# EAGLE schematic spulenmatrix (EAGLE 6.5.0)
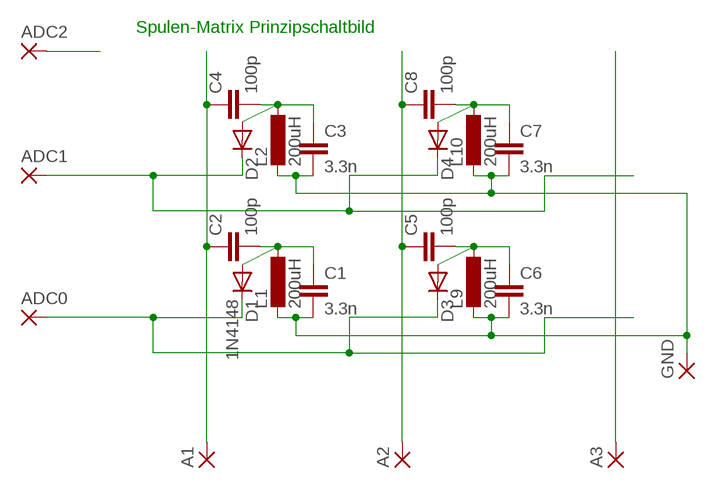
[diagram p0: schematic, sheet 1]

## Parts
A1  WIREPAD2,15/1,0  [2,15/1,0]
A2  WIREPAD2,15/1,0  [2,15/1,0]
A3  WIREPAD2,15/1,0  [2,15/1,0]
ADC0  WIREPAD2,15/1,0  [2,15/1,0]
ADC1  WIREPAD2,15/1,0  [2,15/1,0]
ADC2  WIREPAD2,15/1,0  [2,15/1,0]
C1  3.3n  C2,5-3  [C2.5-3]
C2  100p  C2,5-3  [C2.5-3]
C3  3.3n  C2,5-3  [C2.5-3]
C4  100p  C2,5-3  [C2.5-3]
C5  100p  C2,5-3  [C2.5-3]
C6  3.3n  C2,5-3  [C2.5-3]
C7  3.3n  C2,5-3  [C2.5-3]
C8  100p  C2,5-3  [C2.5-3]
D1  1N4148  1N4148DO35-7  [DO35-7]
D2  1N4148DO35-7  [DO35-7]
D3  1N4148DO35-7  [DO35-7]
D4  1N4148DO35-7  [DO35-7]
GND  WIREPAD2,15/1,0  [2,15/1,0]
L1  200uH  L-EU0204/5  [0204/5]
L2  200uH  L-EU0204/5  [0204/5]
L9  200uH  L-EU0204/5  [0204/5]
L10  200uH  L-EU0204/5  [0204/5]

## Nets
N$1: ADC0.1(P) D1.C D3.C
N$2 [dick]: A1.1(P) C2.1 C4.1
N$3 [dick]: A2.1(P) C5.1 C8.1
N$4: C3.1 C4.2 D2.A L2.1
N$5: C5.2 C6.1 D3.A L9.1
N$6: ADC1.1(P) D2.C D4.C
N$7: ADC2.1(P)
N$9: A3.1(P)
N$11: C1.1 C2.2 D1.A L1.1
N$12: C1.2 C3.2 C6.2 C7.2 GND.1(P) L1.2 L2.2 L9.2 L10.2
N$13: C7.1 C8.2 D4.A L10.1

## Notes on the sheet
- Spulen-Matrix Prinzipschaltbild

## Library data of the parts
A1-A3 ADC0 ADC1 ADC2 GND = wirepad:WIREPAD: Wire PAD connect wire on PCB
C1-C8 = capacitor-wima:C: CAPACITOR
D1-D4 = diode:1N4148: DIODE
L1 L2 L9 L10 = rcl:L-EU: INDUCTOR, European symbol

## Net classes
1 dick: width 0.508 mm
